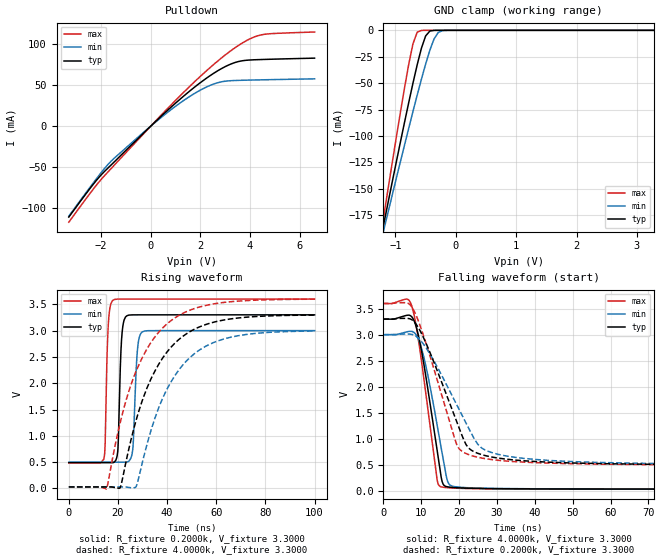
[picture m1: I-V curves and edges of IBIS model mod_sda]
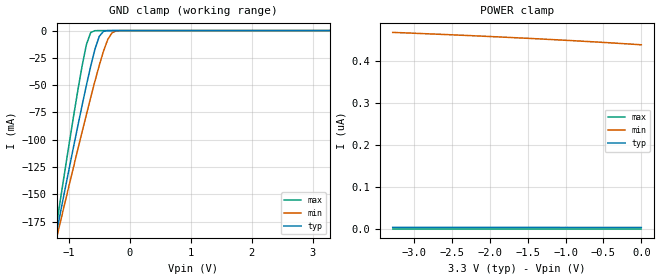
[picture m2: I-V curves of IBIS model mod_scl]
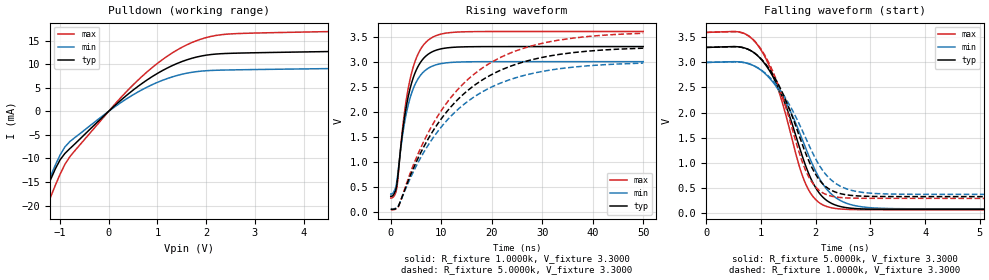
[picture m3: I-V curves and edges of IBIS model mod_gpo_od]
| IBIS (I/O, Buffer, Information, Specification) Model, officially
| electronic behavioral standard for Buffer structures of digital pins.
[IBIS ver]  4.0
[File name] st25dv04kc_so8_3v3.ibs
[File Rev]  1.0
[Date]   19 March 2024
[Notes]
   (Note1)  This IBIS model includes the SO8 package data
   (Note2)  This IBIS model has some Notes about the non-monotonicity
   of the I-V curves, but they are not indicative of problems
   inside the model;
[Disclaimer]
   Customers are solely responsible for all aspects of their
   own product designs or applications using this IBIS Model.
   STMicroelectronics assumes no liability for Custmer Designs
   and applications associated to this IBIS Model.
   In the use of this IBIS Model Customer shall not modify,
   disassemble, alter this Model in whole or in part.
   If Customers do not accept these terms, the IBIS Model
   may not be used. For any problems or modifications please
   contact STMicroelectronics (www.st.com).
[Copyright] (c) 2024 STMicroelectronics
|   Component ST25DV04K
[Component] ST25DV04K
[Manufacturer] STMicroelectronics
[Package]
| variable  typ   min   max
R_pkg   0.0   0.0   0.0
L_pkg   0.0H   0.0H   0.0H
C_pkg   0.0F   0.0F   0.0F
[Pin]  signal_name   model_name   R_pin   L_pin   C_pin
1   VEH   NC   0.0   0.0   0.0
2   AC0   NC   0.0   0.0   0.0
3   AC1   NC   0.0   0.0   0.0
4   VSS   GND   130.95m   2.182nH   0.287pF
5   SDA   mod_sda   130.79m   2.182nH   0.286pF
6   SCL   mod_scl   85.32m   1.589nH   0.354pF
7   GPO   mod_gpo_od   84.54m   1.583nH   0.355pF
8   VCC   POWER   124.14m   2.142nH   0.284pF
| Models and submodels in the file (3): mod_sda (I/O_open_drain), mod_scl (Input), mod_gpo_od (Open_drain)
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|   Model mod_sda
[Model]   mod_sda
Model_type I/O_open_drain
Polarity   Non-Inverting
Enable   Active-Low
Vinl   =   0.825V
Vinh   =   2.457V
Vmeas  =   1.650V
Cref   =   30pF
Rref   =   4.0k
Vref   =   3.30V
C_comp   3.063pF   2.925pF   3.207pF
[Model Spec]
Vinl   0.825V   0.750V   0.900V
Vinh   2.475V   2.250V   2.700V
Vmeas   1.650V   1.500V   1.800V
[Temperature Range]   25.0000   85.0000   -40.0000
[Voltage Range]   3.3000V   3.0000V   3.6000V
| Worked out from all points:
|   slope of the pulldown table from 0 to 0.495 V, typ, clamps not added: 34.9 ohm
|   GND clamp passes 1 mA (typ) near -0.43 V on its own axis
|   rising waveform, R_fixture 0.2000k, V_fixture 3.3000: 20-80 % time 1.1ns typ, 1.34ns min, 981ps max; typ from 0.49 V to 3.3 V
|   rising waveform, R_fixture 4.0000k, V_fixture 3.3000: 20-80 % time 16.7ns typ, 16.8ns min, 16.6ns max; typ from 0.028 V to 3.3 V
|   falling waveform, R_fixture 4.0000k, V_fixture 3.3000: 20-80 % time 4.19ns typ, 4.54ns min, 3.92ns max; typ from 3.3 V to 0.028 V
|   falling waveform, R_fixture 0.2000k, V_fixture 3.3000: 20-80 % time 8.96ns typ, 10.6ns min, 7.75ns max; typ from 3.3 V to 0.495 V
[Pulldown]
|Voltage   I(typ)   I(min)   I(max)
-3.3V     -110.9mA   -109.8mA   -117.1mA
-2.2V     -66.52mA   -64.63mA   -72.36mA
-1.6V     -47.45mA   -42.8mA    -51.82mA
500mV     14.34mA    12.55mA    15.93mA
1.2V      33.37mA    28.63mA    37.49mA
1.9V      50.74mA    42.29mA    57.94mA
2.5V      63.75mA    50.98mA    74.29mA
3.1V      74.05mA    55.15mA    89.1mA
3.6V      79.24mA    55.88mA    99.71mA
4.1V      80.83mA    56.25mA    107.9mA
4.8V      81.56mA    56.69mA    112.7mA
6.6V      82.93mA    57.69mA    114.7mA
[GND_clamp]
|Voltage   I(typ)   I(min)   I(max)
-3.3V     -795.2mA   -697.3mA   -961.3mA
-1.27V    -204.7mA   -206.9mA   -203.5mA
-1.2V     -184.8mA   -190.3mA   -177.9mA
-1.13V    -165mA     -173.8mA   -152.6mA
-780mV    -68.24mA   -92.51mA   -32.05mA
-710mV    -49.95mA   -76.74mA   -12.73mA
-640mV    -32.56mA   -61.26mA   -1.741mA
-500mV    -5.297mA   -31.88mA   -2.458uA
-360mV    -51.44uA   -8.102mA   -2.781nA
-290mV    -3.647uA   -1.956mA   -95.8pA
-220mV    -258.4nA   -266.7uA   -5.411pA
3.28V     2.763nA    443nA      9.537pA
[Ramp]
| variable   typ   min   max
dV/dt_r   1.1470/1.1762n   0.9724/1.4202n   1.3136/1.0919n
dV/dt_f   1.1287/16.5685n  0.9476/20.4603n  1.3005/13.8174n
R_load = 50.0000
[Rising Waveform]
R_fixture= 0.2000k
V_fixture= 3.3000
V_fixture_min= 3.0000
V_fixture_max= 3.6000
|time   V(typ)   V(min)   V(max)
0s        489.7mV    498.4mV    488.3mV
14.26ns   489.7mV    498.4mV    564.7mV
16.02ns   489.7mV    498.4mV    3.085V
18.04ns   490mV      498.4mV    3.58V
19.86ns   683.3mV    498.4mV    3.599V
21.46ns   2.83V      498.4mV    3.6V
23.52ns   3.279V     499.1mV    3.6V
26.02ns   3.299V     741.3mV    3.6V
29.96ns   3.3V       2.978V     3.6V
100ns     3.3V       3V         3.6V
[Rising Waveform]
R_fixture= 4.0000k
V_fixture= 3.3000
V_fixture_min= 3.0000
V_fixture_max= 3.6000
|time   V(typ)   V(min)   V(max)
0s        28.03mV    28.81mV    27.72mV
15.34ns   28.03mV    28.81mV    -8.923mV
20.92ns   14.59mV    28.82mV    1.252V
27.38ns   1.295V     32.77mV    2.229V
31.84ns   1.913V     844.9mV    2.656V
35.04ns   2.232V     1.337V     2.882V
41.44ns   2.678V     2.014V     3.185V
49.44ns   2.985V     2.495V     3.392V
60.64ns   3.179V     2.804V     3.521V
100ns     3.296V     2.993V     3.597V
[Falling Waveform]
R_fixture= 4.0000k
V_fixture= 3.3000
V_fixture_min= 3.0000
V_fixture_max= 3.6000
|time   V(typ)   V(min)   V(max)
0s        3.3V       3V         3.6V
6.2ns     3.373V     3.055V     3.685V
7.6ns     3.335V     3.061V     3.527V
8.92ns    3.084V     2.962V     3.056V
10.6ns    2.47V      2.592V     2.205V
14.08ns   823mV      1.309V     256.1mV
15.04ns   356.9mV    913mV      78.04mV
16.96ns   72.52mV    179.2mV    55.46mV
19.06ns   56.59mV    73.76mV    46.63mV
100ns     28.38mV    29.32mV    27.97mV
[Falling Waveform]
R_fixture= 0.2000k
V_fixture= 3.3000
V_fixture_min= 3.0000
V_fixture_max= 3.6000
|time   V(typ)   V(min)   V(max)
0s        3.3V       3V         3.6V
6.16ns    3.314V     3.013V     3.613V
8.02ns    3.257V     2.994V     3.47V
11.92ns   2.724V     2.673V     2.68V
19.3ns    1.335V     1.66V      899.5mV
21.82ns   886.4mV    1.298V     713.3mV
24.22ns   738.6mV    969.6mV    653.9mV
26.1ns    689.3mV    812.9mV    624.5mV
34.5ns    589.7mV    642.9mV    558.4mV
100ns     495.1mV    506.5mV    492.1mV
|   Model mod_scl
[Model]   mod_scl
Model_type Input
Vinl   =   0.825V
Vinh   =   2.475V
C_comp   2.118pF   2.024pF   2.219pF
[Model Spec]
Vinl   0.825V   0.750V   0.900V
Vinh   2.475V   2.250V   2.700V
[Temperature Range]  25.0000   85.0000   -40.0000
[Voltage Range]   3.3000V   3.0000V   3.6000V
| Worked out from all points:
|   GND clamp passes 1 mA (typ) near -0.43 V on its own axis
[GND_clamp]
|Voltage   I(typ)   I(min)   I(max)
-3.3V     -795.2mA   -697.3mA   -961.3mA
-1.27V    -204.7mA   -206.9mA   -203.5mA
-1.2V     -184.8mA   -190.3mA   -177.9mA
-1.13V    -165mA     -173.8mA   -152.6mA
-780mV    -68.24mA   -92.51mA   -32.05mA
-710mV    -49.95mA   -76.74mA   -12.73mA
-640mV    -32.56mA   -61.26mA   -1.741mA
-500mV    -5.297mA   -31.88mA   -2.458uA
-360mV    -51.44uA   -8.102mA   -2.781nA
-290mV    -3.647uA   -1.956mA   -95.8pA
-220mV    -258.4nA   -266.7uA   -5.411pA
3.28V     2.763nA    443nA      9.537pA
[POWER_clamp]
|Voltage   I(typ)   I(min)   I(max)
-3.28V    3.192nA    469.4nA    17.22pA
-3.16V    3.179nA    468.6nA    16.97pA
-2.24V    3.077nA    461.6nA    15.02pA
-1.48V    2.983nA    455.1nA    13.41pA
-800mV    2.89nA     448.6nA    11.95pA
-440mV    2.837nA    444.8nA    11.18pA
-120mV    2.786nA    441.2nA    10.49pA
0V        2.766nA    439.7nA    10.23pA
|   Model mod_gpo_od
[Model]   mod_gpo_od
Model_type Open_drain
Polarity   Non-Inverting
Enable   Active-Low
Vmeas  =   1.650V
Cref   =   30.0pF
Rref   =   5.0k
Vref   =   3.30V
C_comp   2.219pF   2.119pF   2.324pF
[Model Spec]
Vmeas   1.650V   1.500V   1.800V
[Temperature Range]  25.0000   85.0000   -40.0000
[Voltage Range]   3.3000V   3.0000V   3.6000V
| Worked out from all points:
|   slope of the pulldown table from 0 to 0.495 V, typ, clamps not added: 112 ohm
|   rising waveform, R_fixture 1.0000k, V_fixture 3.3000: 20-80 % time 2.94ns typ, 2.95ns min, 2.93ns max; typ from 0.321 V to 3.3 V
|   rising waveform, R_fixture 5.0000k, V_fixture 3.3000: 20-80 % time 14.2ns typ, 14.3ns min, 14.2ns max; typ from 0.067 V to 3.27 V
|   falling waveform, R_fixture 5.0000k, V_fixture 3.3000: 20-80 % time 648ps typ, 737ps min, 580ps max; typ from 3.3 V to 0.067 V
|   falling waveform, R_fixture 1.0000k, V_fixture 3.3000: 20-80 % time 676ps typ, 762ps min, 609ps max; typ from 3.3 V to 0.321 V
[Pulldown]
|Voltage   I(typ)   I(min)   I(max)
-3.3V     -75.45mA   -74.49mA   -76.82mA
-1.5V     -22.59mA   -21.88mA   -26.22mA
-1.4V     -19.85mA   -19.16mA   -23.57mA
-1.3V     -17.19mA   -16.5mA    -20.94mA
-1.1V     -12.3mA    -11.5mA    -15.8mA
-900mV    -8.956mA   -7.571mA   -11.25mA
-800mV    -7.944mA   -6.452mA   -9.669mA
700mV     6.016mA    4.65mA     7.545mA
1.3V      9.659mA    7.269mA    12.34mA
1.8V      11.48mA    8.399mA    14.95mA
2.5V      12.28mA    8.761mA    16.4mA
6.6V      13.62mA    9.931mA    17.93mA
[Ramp]
| variable   typ   min   max
dV/dt_r   0.3700/0.9678n   0.2632/0.9714n  0.4955/0.9715n
dV/dt_f   0.3698/0.8570n   0.2629/0.8545n  0.4962/0.8629n
R_load = 50.0000
[Rising Waveform]
R_fixture= 1.0000k
V_fixture= 3.3000
V_fixture_min= 3.0000
V_fixture_max= 3.6000
|time   V(typ)   V(min)   V(max)
0s        321.3mV    366.2mV    286.2mV
700ps     376.2mV    427.6mV    333.2mV
1.2ns     554.2mV    619.7mV    490mV
2.6ns     1.812V     1.713V     1.905V
3.3ns     2.232V     2.076V     2.385V
4.1ns     2.57V      2.368V     2.769V
5.7ns     2.959V     2.704V     3.212V
7.9ns     3.18V      2.896V     3.464V
14.3ns    3.294V     2.995V     3.594V
50ns      3.3V       3V         3.6V
[Rising Waveform]
R_fixture= 5.0000k
V_fixture= 3.3000
V_fixture_min= 3.0000
V_fixture_max= 3.6000
|time   V(typ)   V(min)   V(max)
0s        66.67mV    76.48mV    59.08mV
1.55ns    129.5mV    137.5mV    120.8mV
5.45ns    1.09V      1.003V     1.178V
9.65ns    1.815V     1.657V     1.973V
13.65ns   2.284V     2.081V     2.487V
18.05ns   2.631V     2.394V     2.868V
23.7ns    2.909V     2.646V     3.172V
30.7ns    3.099V     2.818V     3.38V
39.05ns   3.209V     2.918V     3.501V
50ns      3.268V     2.971V     3.565V
[Falling Waveform]
R_fixture= 5.0000k
V_fixture= 3.3000
V_fixture_min= 3.0000
V_fixture_max= 3.6000
|time   V(typ)   V(min)   V(max)
0s        3.3V       3V         3.6V
645ps     3.304V     3.007V     3.598V
945ps     3.131V     2.889V     3.343V
1.365ns   2.387V     2.379V     2.297V
1.815ns   943.9mV    1.299V     582.8mV
2.055ns   409.1mV    711.5mV    209.3mV
2.295ns   183.4mV    364mV      96.95mV
2.685ns   85.97mV    149.3mV    63.02mV
3.375ns   67.44mV    82.49mV    59.15mV
15ns      66.67mV    76.48mV    59.08mV
[Falling Waveform]
R_fixture= 1.0000k
V_fixture= 3.3000
V_fixture_min= 3.0000
V_fixture_max= 3.6000
|time   V(typ)   V(min)   V(max)
0s        3.3V       3V         3.6V
615ps     3.307V     3.009V     3.604V
945ps     3.136V     2.892V     3.352V
1.365ns   2.463V     2.429V     2.408V
1.845ns   1.112V     1.426V     779.4mV
2.085ns   631.1mV    914.8mV    428.5mV
2.325ns   427.9mV    616.8mV    322.3mV
2.715ns   339.2mV    431.1mV    290mV
3.405ns   322mV      371.8mV    286.3mV
15ns      321.3mV    366.2mV    286.2mV
